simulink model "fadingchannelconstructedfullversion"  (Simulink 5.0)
settings: Solver=ode5  StartTime=0.0  StopTime=10.0  RelTol=1e-3
libraries: commnoisgen2 x2, dspstat3 x2, simulink x2, dspxfrm3 x1

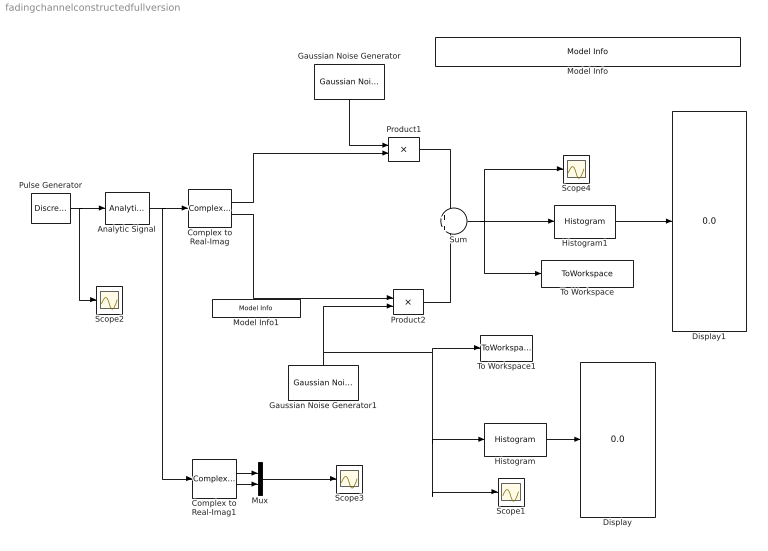
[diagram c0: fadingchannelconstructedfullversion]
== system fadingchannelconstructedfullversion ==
  Analytic Signal : dspxfrm3/Analytic Signal  N=100
  Complex to Real-Imag : ComplexToRealImag
  Complex to Real-Imag1 : ComplexToRealImag
  Display : Display
  Display1 : Display
  Gaussian Noise Generator : commnoisgen2/Gaussian Noise Generator  Orientation=down  m=0  d=0.5  s=41  Ts=.0002  frameBased=off  sampPerFrame=1  orient=on
  Gaussian Noise Generator1 : commnoisgen2/Gaussian Noise Generator  Orientation=up  m=0  d=0.5  s=41  Ts=.0002  frameBased=off  sampPerFrame=1  orient=off
  Histogram : dspstat3/Histogram  umin=-1.5  umax=1.5  nbins=9  normalized=on  run=on  reset=off  trigtype=Either edge
  Histogram1 : dspstat3/Histogram  umin=-1.45  umax=1.45  nbins=13  normalized=on  run=on  reset=off  trigtype=Either edge
  Model Info : simulink/Model-Wide Utilities/Model Info  InitialBlockCM=None  BlockCM=None  Frame=on  DisplayStringWithTags=Constructed Rayleigh Fading Channel  HorizontalTextAlignment=Center  LeftAlignmentValue=0.5  SourceBlockDiagram=fadingchannelconstructedfullversion  TagMaxNumber=20
  Model Info1 : simulink/Model-Wide Utilities/Model Info  InitialBlockCM=None  BlockCM=None  Frame=on  DisplayStringWithTags=Hilbert Transformed  HorizontalTextAlignment=Center  LeftAlignmentValue=0.5  SourceBlockDiagram=fadingchannelconstructedfullversion  TagMaxNumber=20
  Mux : Mux  Inputs=2
  Product1 : Product  ShowAdditionalParam=on
  Product2 : Product
  Pulse Generator : DiscretePulseGenerator  SampleTime=.0002
  Scope{1..4} (4 alike) : Scope
  Sum : Sum  Inputs=+|+  ShowAdditionalParam=on
  To Workspace : ToWorkspace  VariableName=RayleighPDFOutput  SampleTime=-1  SaveFormat=Structure
  To Workspace1 : ToWorkspace  VariableName=AWGN  SampleTime=-1  SaveFormat=Structure
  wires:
  Product1/1 -> Sum/1
  Product2/1 -> Sum/2
  Gaussian Noise Generator/1 -> Product1/1
  Gaussian Noise Generator1/1 -> Product2/2, Scope1/1, Histogram/1, To Workspace1/1
  Sum/1 -> Scope4/1, To Workspace/1, Histogram1/1
  Complex to Real-Imag/1 -> Product1/2
  Complex to Real-Imag/2 -> Product2/1
  Analytic Signal/1 -> Complex to Real-Imag/1, Complex to Real-Imag1/1
  Pulse Generator/1 -> Analytic Signal/1, Scope2/1
  Complex to Real-Imag1/1 -> Mux/1
  Complex to Real-Imag1/2 -> Mux/2
  Mux/1 -> Scope3/1
  Histogram1/1 -> Display1/1
  Histogram/1 -> Display/1
